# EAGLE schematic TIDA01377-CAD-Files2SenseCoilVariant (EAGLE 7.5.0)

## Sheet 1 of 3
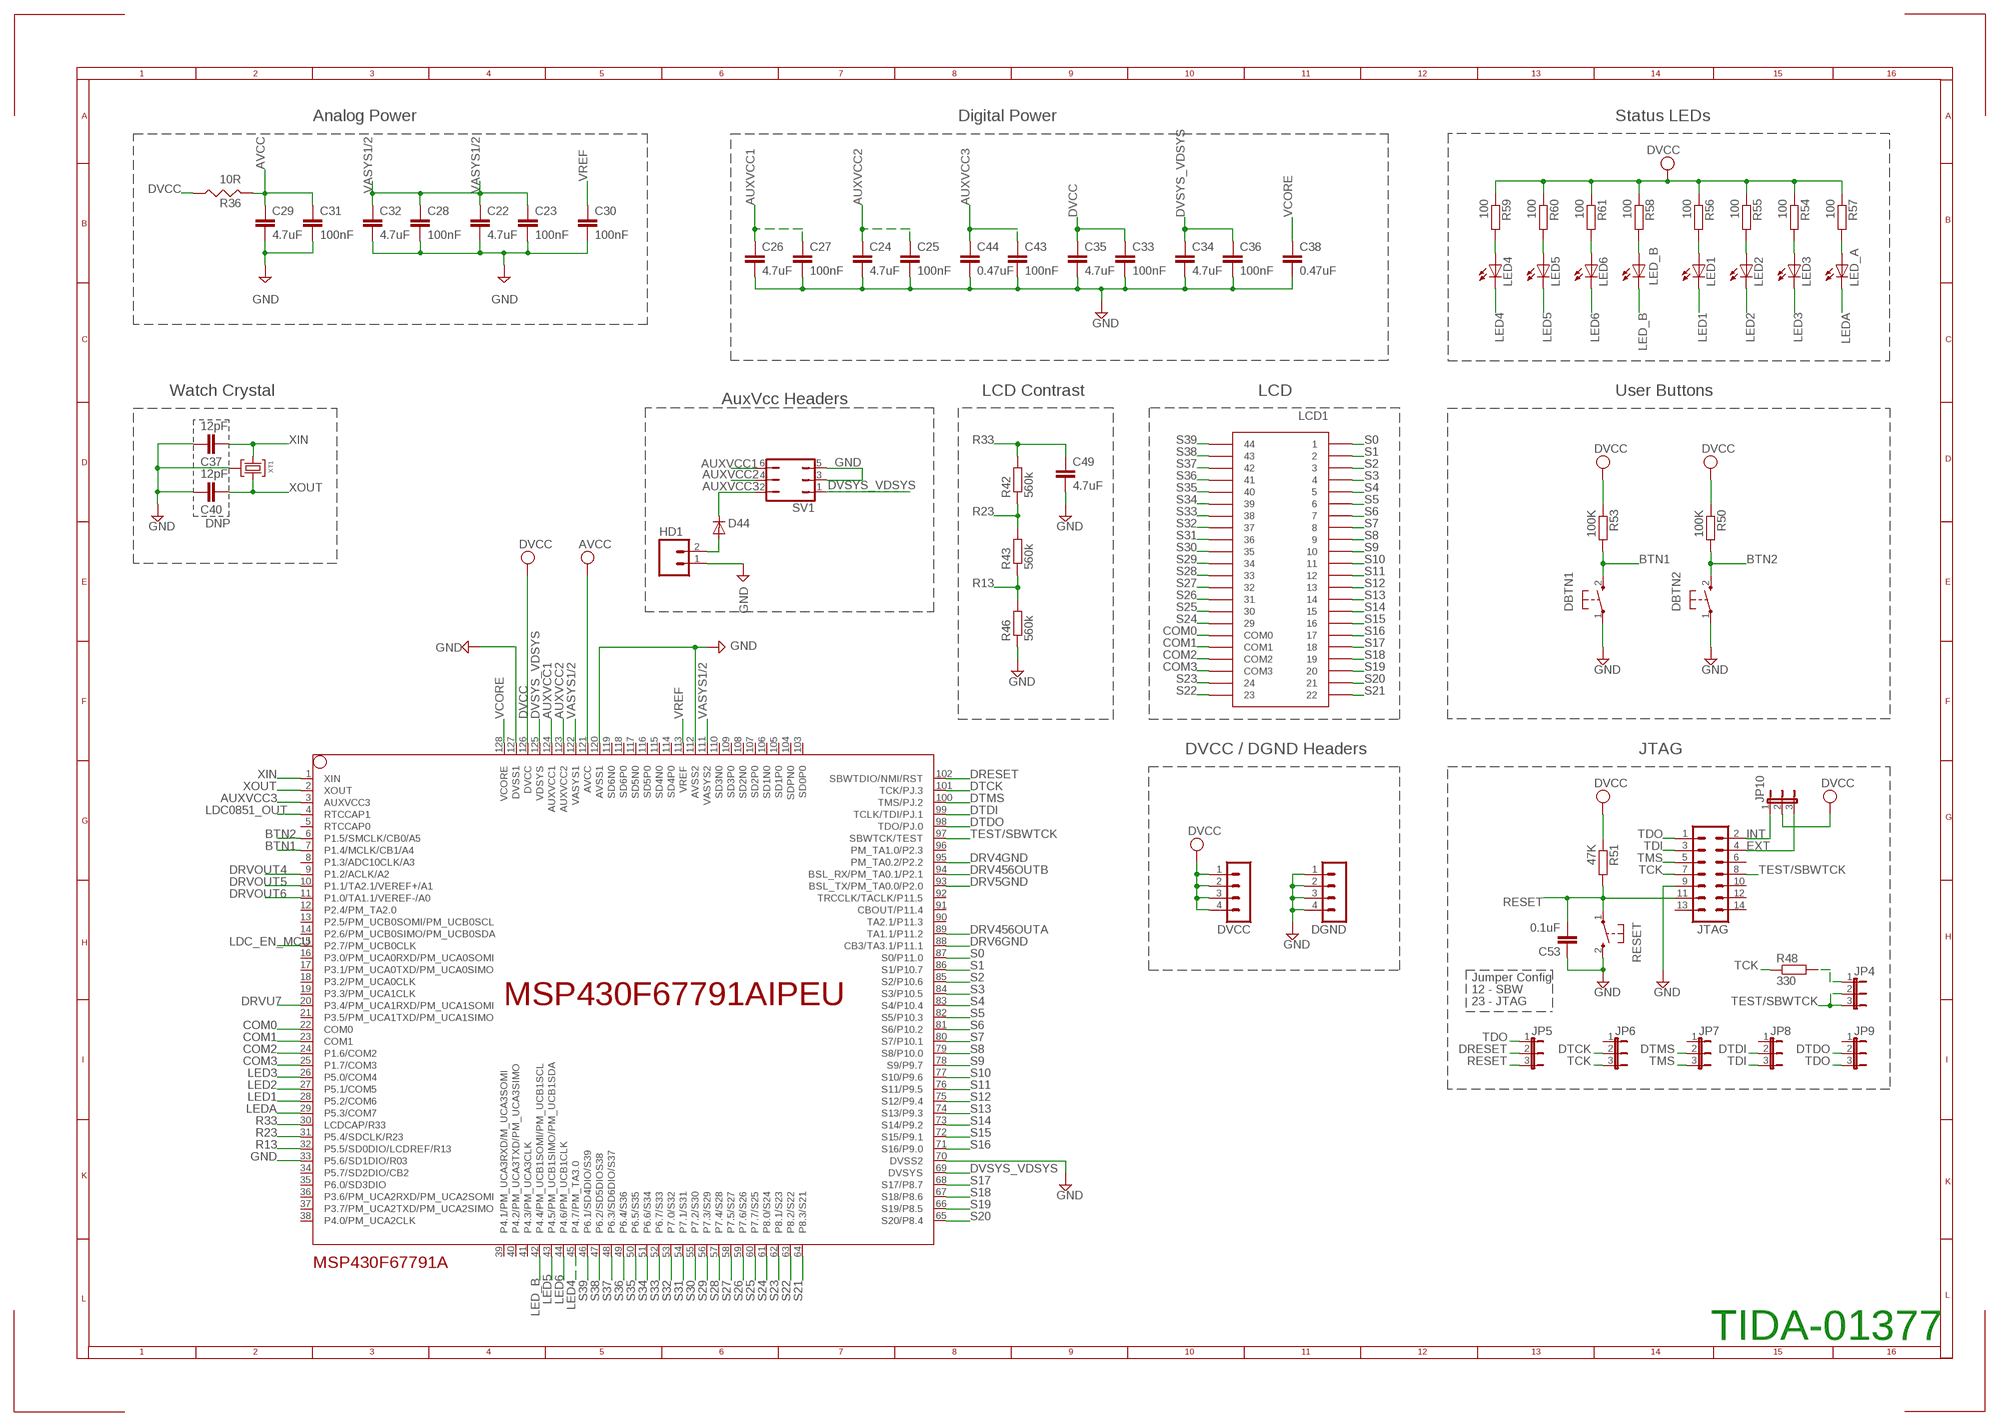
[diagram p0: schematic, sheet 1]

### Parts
C22  4.7uF  C-EUC0603  [C0603]
C23  100nF  C-EUC0603  [C0603]
C24  4.7uF  C-EUC0603  [C0603]
C25  100nF  C-EUC0603  [C0603]
C26  4.7uF  C-EUC0603  [C0603]
C27  100nF  C-EUC0603  [C0603]
C28  100nF  C-EUC0603  [C0603]
C29  4.7uF  C-EUC0603  [C0603]
C30  100nF  C-EUC0603  [C0603]
C31  100nF  C-EUC0603  [C0603]
C32  4.7uF  C-EUC0603  [C0603]
C33  100nF  C-EUC0603  [C0603]
C34  4.7uF  C-EUC0603  [C0603]
C35  4.7uF  C-EUC0603  [C0603]
C36  100nF  C-EUC0603  [C0603]
C37  12pF  C-EUC0603  [C0603]
C38  0.47uF  C-EUC0603  [C0603]
C40  12pF  C-EUC0603  [C0603]
C43  100nF  C-EUC0603  [C0603]
C44  0.47uF  C-EUC0603  [C0603]
C49  4.7uF  C-EUC0603  [C0603]
C53  0.1uF  C-EUC0603  [C0603]
D44  PMLL4148  [SOD80C]
DBTN1  PB  [PBTH]
DBTN2  PB  [PBTH]
DGND  MA04-1  [MA04-1]
DVCC  MA04-1  [MA04-1]
HD1  M02PTH  [1X02]
JP4  JP2E  [JP2]
JP5  JP2E  [JP2]
JP6  JP2E  [JP2]
JP7  JP2E  [JP2]
JP8  JP2E  [JP2]
JP9  JP2E  [JP2]
JP10  JP2E  [JP2]
JTAG  ML14  [ML14]
LCD1  TI_160SEG_LCD  [TI_160SEG_LCD]
LED1  LED3MM  [LED3MM]
LED2  LED3MM  [LED3MM]
LED3  LED3MM  [LED3MM]
LED4  LED3MM  [LED3MM]
LED5  LED3MM  [LED3MM]
LED6  LED3MM  [LED3MM]
LED_A  LED3MM  [LED3MM]
LED_B  LED3MM  [LED3MM]
MSP430F67791A  MSP430F6779AIPEU  [PEU128]
R36  10R  RES0805  [R0805]
R42  560k  R-EU_R0603  [R0603]
R43  560k  R-EU_R0603  [R0603]
R46  560k  R-EU_R0603  [R0603]
R48  330  R-EU_R0603  [R0603]
R50  100K  R-EU_R0603  [R0603]
R51  47K  R-EU_R0603  [R0603]
R53  100K  R-EU_R0603  [R0603]
R54  100  R-EU_R0603  [R0603]
R55  100  R-EU_R0603  [R0603]
R56  100  R-EU_R0603  [R0603]
R57  100  R-EU_R0603  [R0603]
R58  100  R-EU_R0603  [R0603]
R59  100  R-EU_R0603  [R0603]
R60  100  R-EU_R0603  [R0603]
R61  100  R-EU_R0603  [R0603]
RESET  PB  [PBTH]
SV1  JP3Q  [JP3Q]
XT1  CM200T  [CM200T]

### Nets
AUXVCC1: C26.1 C27.1 MSP430F67791A.124(AUXVCC1) SV1.6
AUXVCC2: C24.1 C25.1 MSP430F67791A.123(AUXVCC2) SV1.4 ; also sheet 2
AUXVCC3: C43.1 C44.1 D44.C MSP430F67791A.3(AUXVCC3) SV1.2
AVCC: C29.1 C31.1 MSP430F67791A.121(AVCC) R36.2
BTN1: DBTN1.2(S) MSP430F67791A.7(P1.4/MCLK/CB1/A4) R53.2
BTN2: DBTN2.2(S) MSP430F67791A.6(P1.5/SMCLK/CB0/A5) R50.2
COM0: LCD1.COM0 MSP430F67791A.22(COM0)
COM1: LCD1.COM1 MSP430F67791A.23(COM1)
COM2: LCD1.COM2 MSP430F67791A.24(P1.6/COM2)
COM3: LCD1.COM3 MSP430F67791A.25(P1.7/COM3)
DRESET: JP5.2 MSP430F67791A.102(SBWTDIO/NMI/RST)
DRV4GND: MSP430F67791A.95(PM_TA0.2/P2.2) ; also sheet 2
DRV5GND: MSP430F67791A.93(BSL_TX/PM_TA0.0/P2.0) ; also sheet 2
DRV6GND: MSP430F67791A.88(CB3/TA3.1/P11.1) ; also sheet 2
DRV456OUTA: MSP430F67791A.89(TA1.1/P11.2) ; also sheet 2
DRV456OUTB: MSP430F67791A.94(BSL_RX/PM_TA0.1/P2.1) ; also sheet 2
DRVOUT4: MSP430F67791A.9(P1.2/ACLK/A2) ; also sheet 2
DRVOUT5: MSP430F67791A.10(P1.1/TA2.1/VEREF+/A1) ; also sheet 2
DRVOUT6: MSP430F67791A.11(P1.0/TA1.1/VEREF-/A0) ; also sheet 2
DRVU7: MSP430F67791A.20(P3.4/PM_UCA1RXD/PM_UCA1SOMI) ; also sheet 2
DTCK: JP6.2 MSP430F67791A.101(TCK/PJ.3)
DTDI: JP8.2 MSP430F67791A.99(TCLK/TDI/PJ.1)
DTDO: JP9.2 MSP430F67791A.98(TDO/PJ.0)
DTMS: JP7.2 MSP430F67791A.100(TMS/PJ.2)
DVCC: C33.1 C35.1 DVCC.1 DVCC.2 DVCC.3 DVCC.4 JP10.2 MSP430F67791A.126(DVCC) R36.1 R50.1 R51.1 R53.1 R54.1 R55.1 R56.1 R57.1 R58.1 R59.1 R60.1 R61.1 ; also sheet 2
DVSYS_VDSYS: C34.1 C36.1 MSP430F67791A.69(DVSYS) MSP430F67791A.125(VDSYS) SV1.1 ; also sheet 2,3
EXT: JP10.3 JTAG.4
GND: C22.2 C23.2 C24.2 C25.2 C26.2 C27.2 C28.2 C29.2 C30.2 C31.2 C32.2 C33.2 C34.2 C35.2 C36.2 C37.2 C38.2 C40.2 C43.2 C44.2 C49.2 C53.1 DBTN1.1(P) DBTN2.1(P) DGND.1 DGND.2 DGND.3 DGND.4 HD1.1 JTAG.9 MSP430F67791A.33(P5.6/SD1DIO/R03) MSP430F67791A.70(DVSS2) MSP430F67791A.112(AVSS2) MSP430F67791A.120(AVSS1) MSP430F67791A.127(DVSS1) R46.1 RESET.2(S) SV1.3 SV1.5 XT1.P3 ; also sheet 2,3
INT: JP10.1 JTAG.2
LDC0851_OUT: MSP430F67791A.4(RTCCAP1) ; also sheet 3
LDC_EN_MCU: MSP430F67791A.15(P2.7/PM_UCB0CLK) ; also sheet 3
LED1: LED1.K(C) MSP430F67791A.28(P5.2/COM6)
LED2: LED2.K(C) MSP430F67791A.27(P5.1/COM5)
LED3: LED3.K(C) MSP430F67791A.26(P5.0/COM4)
LED4: LED4.K(C) MSP430F67791A.45(P4.7/PM_TA3.0)
LED5: LED5.K(C) MSP430F67791A.43(P4.5/PM_UCB1SIMO/PM_UCB1SDA)
LED6: LED6.K(C) MSP430F67791A.44(P4.6/PM_UCB1CLK)
LED_B: LED_B.K(C) MSP430F67791A.42(P4.4/PM_UCB1SOMI/PM_UCB1SCL)
LEDA: LED_A.K(C) MSP430F67791A.29(P5.3/COM7)
N$4: LED1.A R56.2
N$7: LED2.A R55.2
N$10: JP4.1 R48.2
N$18: D44.A HD1.2
N$21: LED4.A R59.2
N$27: LED5.A R60.2
N$30: LED3.A R54.2
N$36: LED6.A R61.2
N$44: LED_B.A R58.2
N$46: LED_A.A R57.2
R13: MSP430F67791A.32(P5.5/SD0DIO/LCDREF/R13) R43.1 R46.2
R23: MSP430F67791A.31(P5.4/SDCLK/R23) R42.1 R43.2
R33: C49.1 MSP430F67791A.30(LCDCAP/R33) R42.2
RESET: C53.2 JP5.3 JTAG.11 R51.2 RESET.1(P)
S0: LCD1.1 MSP430F67791A.87(S0/P11.0)
S1: LCD1.2 MSP430F67791A.86(S1/P10.7)
S2: LCD1.3 MSP430F67791A.85(S2/P10.6)
S3: LCD1.4 MSP430F67791A.84(S3/P10.5)
S4: LCD1.5 MSP430F67791A.83(S4/P10.4)
S5: LCD1.6 MSP430F67791A.82(S5/P10.3)
S6: LCD1.7 MSP430F67791A.81(S6/P10.2)
S7: LCD1.8 MSP430F67791A.80(S7/P10.1)
S8: LCD1.9 MSP430F67791A.79(S8/P10.0)
S9: LCD1.10 MSP430F67791A.78(S9/P9.7)
S10: LCD1.11 MSP430F67791A.77(S10/P9.6)
S11: LCD1.12 MSP430F67791A.76(S11/P9.5)
S12: LCD1.13 MSP430F67791A.75(S12/P9.4)
S13: LCD1.14 MSP430F67791A.74(S13/P9.3)
S14: LCD1.15 MSP430F67791A.73(S14/P9.2)
S15: LCD1.16 MSP430F67791A.72(S15/P9.1)
S16: LCD1.17 MSP430F67791A.71(S16/P9.0)
S17: LCD1.18 MSP430F67791A.68(S17/P8.7)
S18: LCD1.19 MSP430F67791A.67(S18/P8.6)
S19: LCD1.20 MSP430F67791A.66(S19/P8.5)
S20: LCD1.21 MSP430F67791A.65(S20/P8.4)
S21: LCD1.22 MSP430F67791A.64(P8.3/S21)
S22: LCD1.23 MSP430F67791A.63(P8.2/S22)
S23: LCD1.24 MSP430F67791A.62(P8.1/S23)
S24: LCD1.29 MSP430F67791A.61(P8.0/S24)
S25: LCD1.30 MSP430F67791A.60(P7.7/S25)
S26: LCD1.31 MSP430F67791A.59(P7.6/S26)
S27: LCD1.32 MSP430F67791A.58(P7.5/S27)
S28: LCD1.33 MSP430F67791A.57(P7.4/S28)
S29: LCD1.34 MSP430F67791A.56(P7.3/S29)
S30: LCD1.35 MSP430F67791A.55(P7.2/S30)
S31: LCD1.36 MSP430F67791A.54(P7.1/S31)
S32: LCD1.37 MSP430F67791A.53(P7.0/S32)
S33: LCD1.38 MSP430F67791A.52(P6.7/S33)
S34: LCD1.39 MSP430F67791A.51(P6.6/S34)
S35: LCD1.40 MSP430F67791A.50(P6.5/S35)
S36: LCD1.41 MSP430F67791A.49(P6.4/S36)
S37: LCD1.42 MSP430F67791A.48(P6.3/SD6DIO/S37)
S38: LCD1.43 MSP430F67791A.47(P6.2/SD5DIOS38)
S39: LCD1.44 MSP430F67791A.46(P6.1/SD4DIO/S39)
TCK: JP6.3 JTAG.7 R48.1
TDI: JP8.3 JTAG.3
TDO: JP5.1 JP9.3 JTAG.1
TEST/SBWTCK: JP4.2 JP4.3 JTAG.8 MSP430F67791A.97(SBWTCK/TEST)
TMS: JP7.3 JTAG.5
VASYS1/2: C22.1 C23.1 C28.1 C32.1 MSP430F67791A.111(VASYS2) MSP430F67791A.122(VASYS1)
VCORE: C38.1 MSP430F67791A.128(VCORE)
VREF: C30.1 MSP430F67791A.113(VREF)
XIN: C37.1 MSP430F67791A.1(XIN) XT1.P2
XOUT: C40.1 MSP430F67791A.2(XOUT) XT1.P1
Unconnected: JP6.1 JP7.1 JP8.1 JP9.1 JTAG.6 JTAG.10 JTAG.12 JTAG.13 JTAG.14 MSP430F67791A.5(RTCCAP0) MSP430F67791A.8(P1.3/ADC10CLK/A3) MSP430F67791A.12(P2.4/PM_TA2.0) MSP430F67791A.13(P2.5/PM_UCB0SOMI/PM_UCB0SCL) MSP430F67791A.14(P2.6/PM_UCB0SIMO/PM_UCB0SDA) MSP430F67791A.16(P3.0/PM_UCA0RXD/PM_UCA0SOMI) MSP430F67791A.17(P3.1/PM_UCA0TXD/PM_UCA0SIMO) MSP430F67791A.18(P3.2/PM_UCA0CLK) MSP430F67791A.19(P3.3/PM_UCA1CLK) MSP430F67791A.21(P3.5/PM_UCA1TXD/PM_UCA1SIMO) MSP430F67791A.34(P5.7/SD2DIO/CB2) MSP430F67791A.35(P6.0/SD3DIO) MSP430F67791A.36(P3.6/PM_UCA2RXD/PM_UCA2SOMI) MSP430F67791A.37(P3.7/PM_UCA2TXD/PM_UCA2SIMO) MSP430F67791A.38(P4.0/PM_UCA2CLK) MSP430F67791A.39(P4.1/PM_UCA3RXD/M_UCA3SOMI) MSP430F67791A.40(P4.2/PM_UCA3TXD/PM_UCA3SIMO) MSP430F67791A.41(P4.3/PM_UCA3CLK) MSP430F67791A.90(TA2.1/P11.3) MSP430F67791A.91(CBOUT/P11.4) MSP430F67791A.92(TRCCLK/TACLK/P11.5) MSP430F67791A.96(PM_TA1.0/P2.3) MSP430F67791A.103(SD0P0) MSP430F67791A.104(SDPN0) MSP430F67791A.105(SD1P0) MSP430F67791A.106(SD1N0) MSP430F67791A.107(SD2P0) MSP430F67791A.108(SD2N0) MSP430F67791A.109(SD3P0) MSP430F67791A.110(SD3N0) MSP430F67791A.114(SD4P0) MSP430F67791A.115(SD4N0) MSP430F67791A.116(SD5P0) MSP430F67791A.117(SD5N0) MSP430F67791A.118(SD6P0) MSP430F67791A.119(SD6N0)

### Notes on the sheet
- Analog Power | Digital Power | Status LEDs
- Watch Crystal | LCD Contrast | LCD | User Buttons
- AuxVcc Headers
- DNP
- DVCC / DGND Headers | JTAG
- Jumper Config
- 12 - SBW
- 23 - JTAG
- TIDA-01377

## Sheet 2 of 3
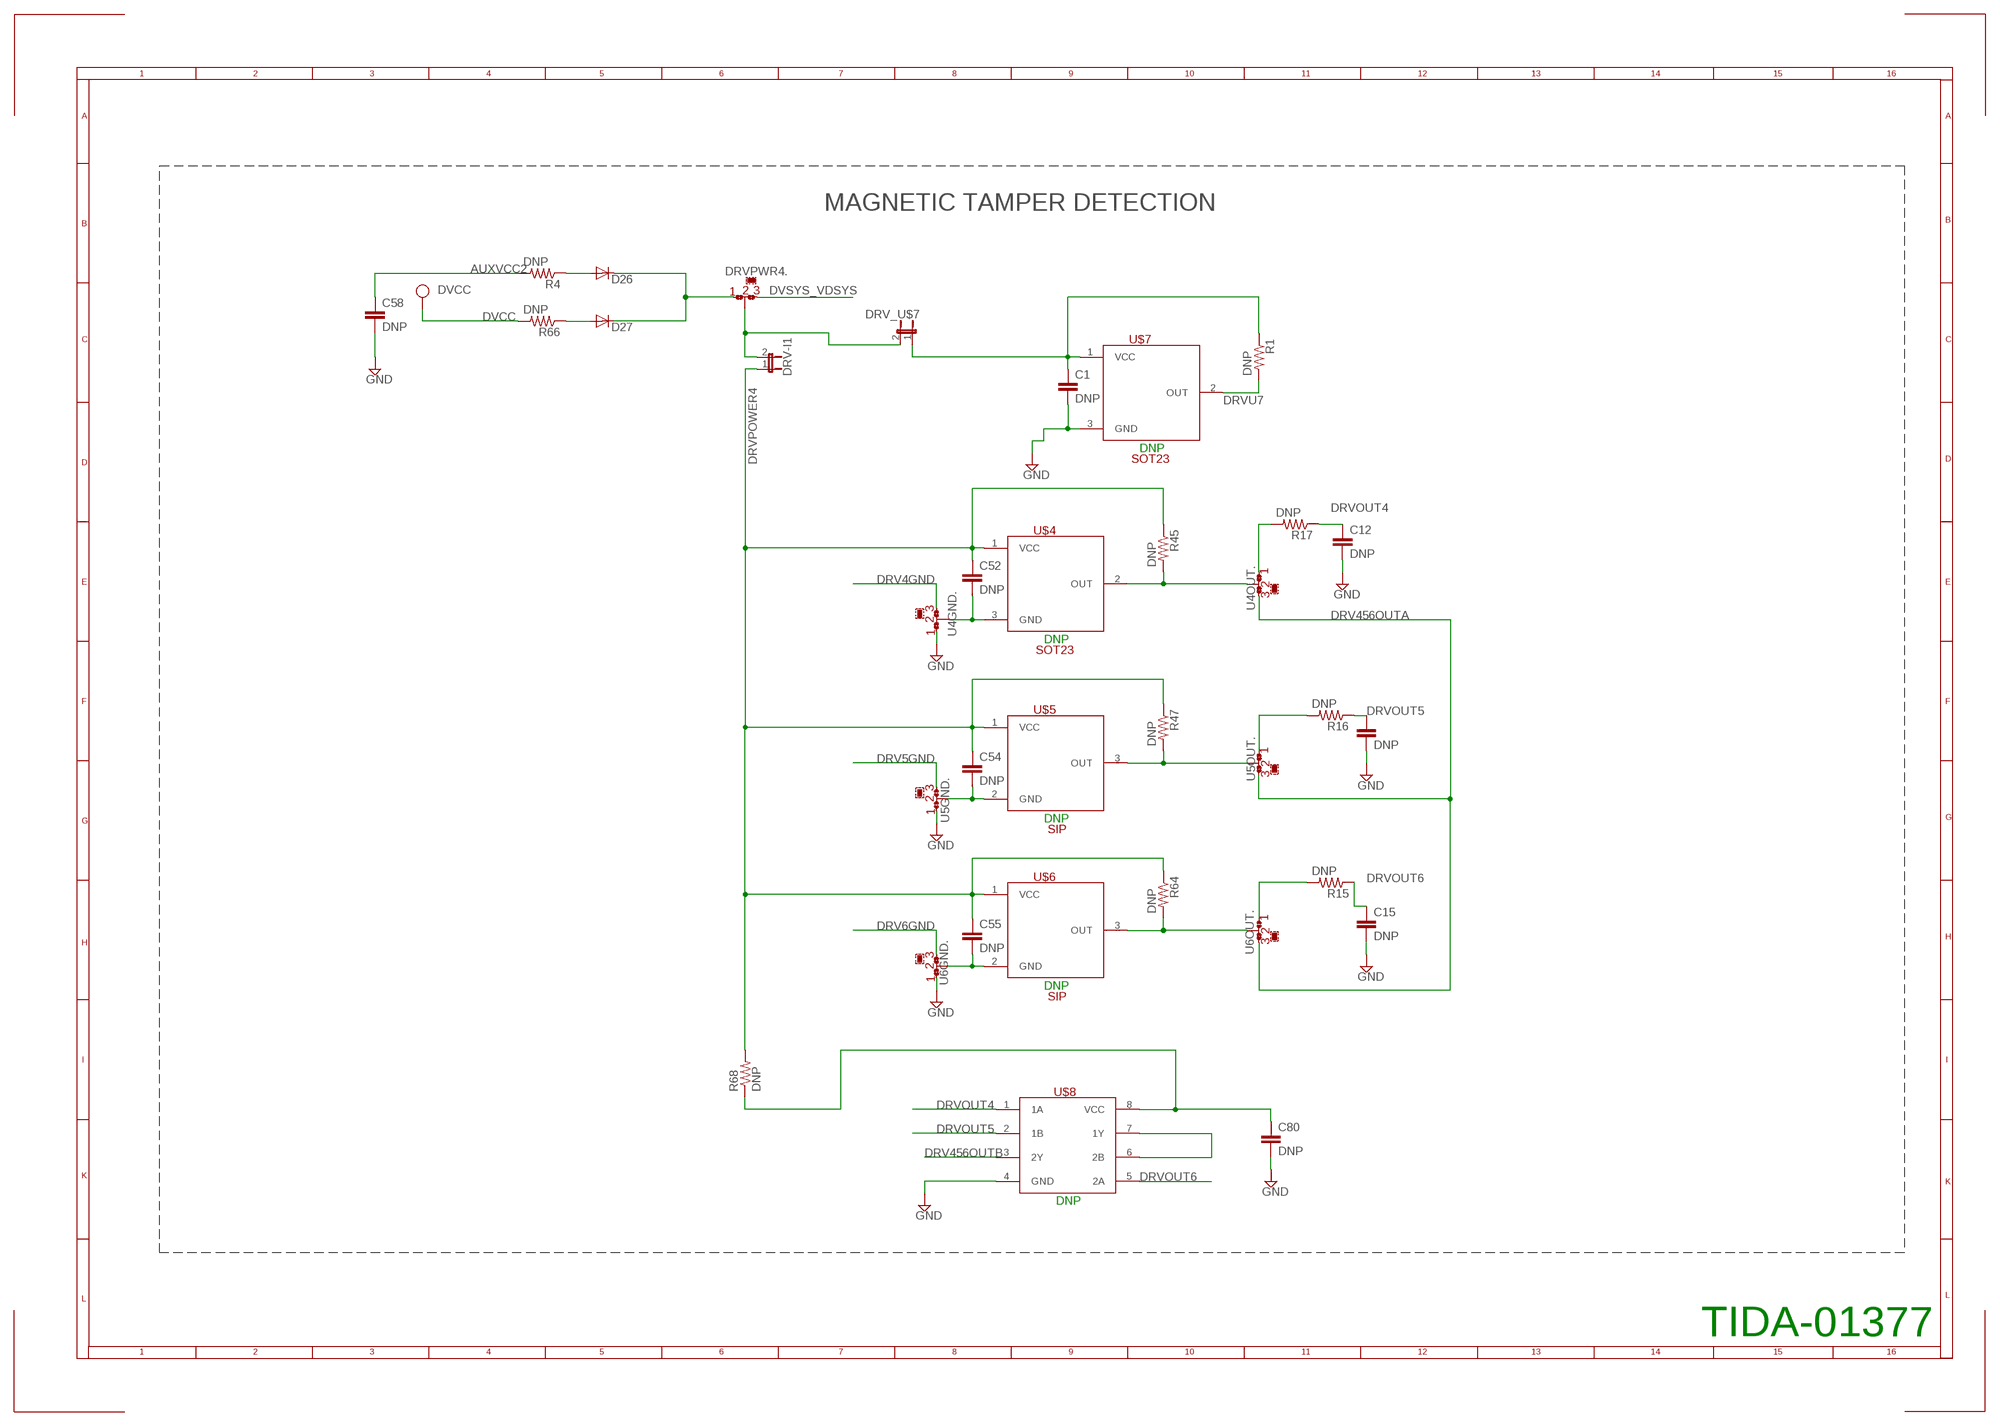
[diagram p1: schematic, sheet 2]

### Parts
C1  DNP  C-EUC0805  [C0805]
C12  DNP  C-EUC0805  [C0805]
C14  DNP  C-EUC0805  [C0805]
C15  DNP  C-EUC0805  [C0805]
C52  DNP  C-EUC0805  [C0805]
C54  DNP  C-EUC0805  [C0805]
C55  DNP  C-EUC0805  [C0805]
C58  DNP  C-EUC0603  [C0603]
C80  DNP  C-EUC0603  [C0603]
D26  PMLL4148  [SOD80C]
D27  PMLL4148  [SOD80C]
DRV-I1  JP1E  [JP1]
DRV_U$7  JP1E  [JP1]
DRVPWR4  0R-JUMPA  [A0R-JMP]
R1  DNP  R-US_R0805  [R0805]
R4  DNP  R-US_R0805  [R0805]
R15  DNP  R-US_R0805  [R0805]
R16  DNP  R-US_R0805  [R0805]
R17  DNP  R-US_R0805  [R0805]
R45  DNP  R-US_R0805  [R0805]
R47  DNP  R-US_R0805  [R0805]
R64  DNP  R-US_R0805  [R0805]
R66  DNP  R-US_R0805  [R0805]
R68  DNP  R-US_R0603  [R0603]
U4GND  0R-JUMPA  [A0R-JMP]
U4OUT  0R-JUMPA  [A0R-JMP]
U5GND  0R-JUMPA  [A0R-JMP]
U5OUT  0R-JUMPA  [A0R-JMP]
U6GND  0R-JUMPA  [A0R-JMP]
U6OUT  0R-JUMPA  [A0R-JMP]
U$4  DRV5033_SOT23  [SOT23]
U$5  DRV5033_SIP  [SIP]
U$6  DRV5033_SIP  [SIP]
U$7  DRV5033_SOT23  [SOT23]
U$8  SN74AUP2G32  [DCU]

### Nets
AUXVCC2: C58.1 R4.2 ; also sheet 1
DRV4GND: U4GND.1 ; also sheet 1
DRV5GND: U5GND.1 ; also sheet 1
DRV6GND: U6GND.1 ; also sheet 1
DRV456OUTA: U4OUT.1 U5OUT.1 U6OUT.1 ; also sheet 1
DRV456OUTB: U$8.3(2Y) ; also sheet 1
DRVOUT4: C12.1 R17.1 U$8.1(1A) ; also sheet 1
DRVOUT5: C14.1 R16.1 U$8.2(1B) ; also sheet 1
DRVOUT6: C15.1 R15.1 U$8.5(2A) ; also sheet 1
DRVPOWER1: C1.1 DRV_U$7.1 R1.1 U$7.1(VCC)
DRVPOWER4: C52.1 C54.1 C55.1 DRV-I1.1 R45.1 R47.1 R64.1 R68.2 U$4.1(VCC) U$5.1(VCC) U$6.1(VCC)
DRVU7: R1.2 U$7.2(OUT) ; also sheet 1
DVCC: R66.2 ; also sheet 1
DVSYS_VDSYS: DRVPWR4.1 ; also sheet 1,3
GND: C1.2 C12.2 C14.2 C15.2 C58.2 C80.2 U4GND.3 U5GND.3 U6GND.3 U$7.3(GND) U$8.4(GND) ; also sheet 1,3
N$17: R17.2 U4OUT.3
N$19: R16.2 U5OUT.3
N$20: R15.2 U6OUT.3
N$24: C52.2 U4GND.2 U$4.3(GND)
N$26: C54.2 U5GND.2 U$5.2(GND)
N$28: C55.2 U6GND.2 U$6.2(GND)
N$41: R45.2 U4OUT.2 U$4.2(OUT)
N$43: R47.2 U5OUT.2 U$5.3(OUT)
N$49: D26.A R4.1
N$50: U$8.6(2B) U$8.7(1Y)
N$51: D27.A R66.1
N$52: D26.C D27.C DRVPWR4.3
N$53: DRV-I1.2 DRV_U$7.2 DRVPWR4.2
N$55: R64.2 U6OUT.2 U$6.3(OUT)
N$58: C80.1 R68.1 U$8.8(VCC)

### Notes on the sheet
- MAGNETIC TAMPER DETECTION
- DNP
- DNP
- DNP
- DNP
- DNP
- TIDA-01377

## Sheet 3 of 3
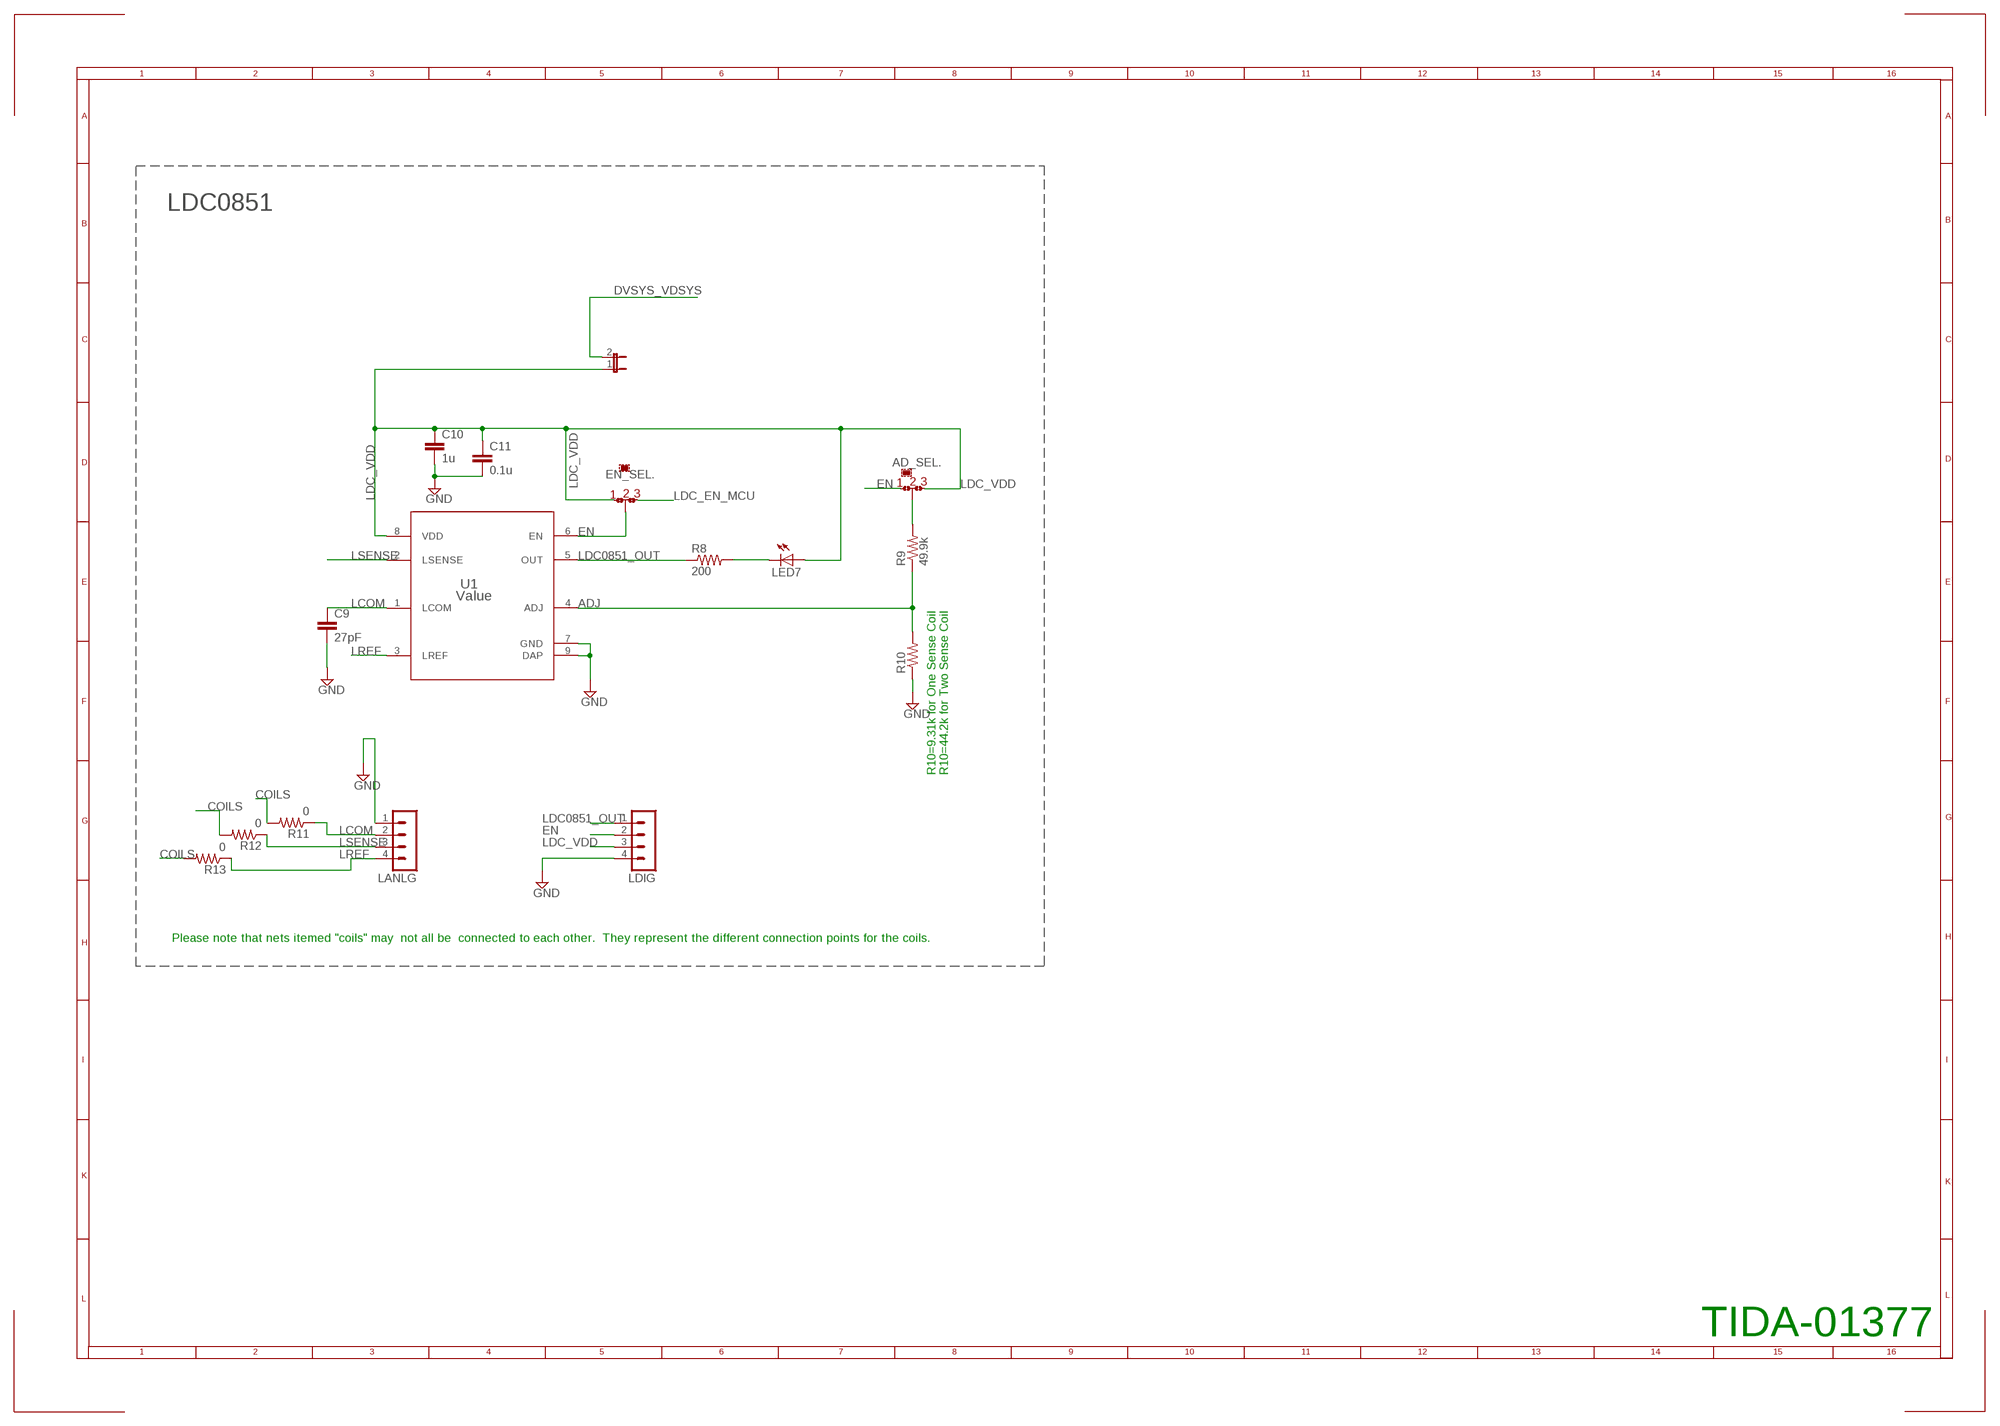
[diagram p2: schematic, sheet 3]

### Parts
AD_SEL  0R-JUMPA  [A0R-JMP]
C9  27pF  C-EUC0603  [C0603]
C10  1u  C-EUC0603  [C0603]
C11  0.1u  C-EUC0402  [C0402]
EN_SEL  0R-JUMPA  [A0R-JMP]
LANLG  MA04-1  [MA04-1]
LDC_PWR  JP1E  [JP1]
LDIG  MA04-1  [MA04-1]
LED7  LEDCHIP-LED0603  [CHIP-LED0603]
R8  200  R-US_R0402  [R0402]
R9  49.9k  R-US_R0603  [R0603]
R10  9.31k(One Sense Coil); 44.2k(Two Sense Coil)  R-US_R0603  [R0603]
R11  0  R-US_R0603  [R0603]
R12  0  R-US_R0603  [R0603]
R13  0  R-US_R0603  [R0603]
U1  Value  LDC0851HDSGR  [DSG0008A]

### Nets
ADJ: R9.1 R10.2 U1.4(ADJ)
COILS: R11.2 R12.2 R13.2
DVSYS_VDSYS: LDC_PWR.2 ; also sheet 1,2
EN: AD_SEL.3 EN_SEL.2 LDIG.2 U1.6(EN)
GND: C9.2 C10.2 C11.2 LANLG.1 LDIG.4 R10.1 U1.7(GND) U1.9(DAP) ; also sheet 1,2
LCOM: C9.1 LANLG.2 R11.1 U1.1(LCOM)
LDC0851_OUT: LDIG.1 R8.1 U1.5(OUT) ; also sheet 1
LDC_EN_MCU: EN_SEL.1 ; also sheet 1
LDC_VDD: AD_SEL.1 C10.1 C11.1 EN_SEL.3 LDC_PWR.1 LDIG.3 LED7.A U1.8(VDD)
LREF: LANLG.4 R13.1 U1.3(LREF)
LSENSE: LANLG.3 R12.1 U1.2(LSENSE)
N$15: LED7.C R8.2
N$16: AD_SEL.2 R9.2

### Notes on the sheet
- LDC0851
- R10=9.31k for One Sense Coil
  R10=44.2k for Two Sense Coil
- Please note that nets itemed "coils" may  not all be  connected to each other.  They represent the different connection points for the coils.
- TIDA-01377

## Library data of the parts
AD_SEL DRVPWR4 EN_SEL U4GND U4OUT U5GND U5OUT U6GND U6OUT = jump-0r-smd:0R-JUMP: SMD 0R 0805 Jumper
C1 C11 C12 C14 C15 C52 C54 C55 = rcl:C-EU: CAPACITOR, European symbol
C9 C10 C22-C38 C40 C43 C44 C49 C53 C58 C80 = resistor:C-EU: CAPACITOR, European symbol
D26 D27 D44 = FE449x EVM:PMLL4148: DIODE
DBTN1 DBTN2 RESET = electricalmeter:PB: OMRON SWITCH
DGND DVCC LANLG LDIG = custom_con-lstb:MA04-1: PIN HEADER; OC_FARNELL: unknown; OC_NEWARK: unknown
DRV-I1 DRV_U$7 LDC_PWR = custom_jumper:JP1E: JUMPER
HD1 = SparkFun:M02: Header 2
JP4-JP10 = custom_jumper:JP2E: JUMPER
JTAG = con-ml:ML14: HARTING; OC_FARNELL: unknown; OC_NEWARK: unknown
LCD1 = Personal:TI_160SEG_LCD
LED1-LED7 LED_A LED_B = led:LED: LED
MSP430F67791A = Personal:MSP430F6779AIPEU: MSP430F6779IPEU
R1 R4 R8 R15-R17 R45 R47 R64 R66 = resistor:R-US_: RESISTOR, American symbol
R9-R13 R68 = rcl:R-US_: RESISTOR, American symbol
R36 = _MSP430:RES
R42 R43 R46 R48 R50 R51 R53-R61 = resistor:R-EU_: RESISTOR, European symbol
SV1 = jumper:JP3Q: JUMPER
U1 = LDC0851:LDC0851HDSGR; ALTERNATEPARTNUMBER: LDC0851DSGT; COMPTYPE: IC; MANUFACTURER: Texas Instruments; MOUNTTYPE: SMT; PACKAGEREFERENCE: DSG0008A; PARTNUMBER: LDC0851DSGR; PIN_COUNT: 9; REFDES: RefDes; TYPE: TYPE
U$4 U$7 = DRVlibrary:DRV5033_SOT23
U$5 U$6 = DRVlibrary:DRV5033_SIP
U$8 = SN74AUP2G32:SN74AUP2G32
XT1 = F20xx PIR Demo & Eval:CM200T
